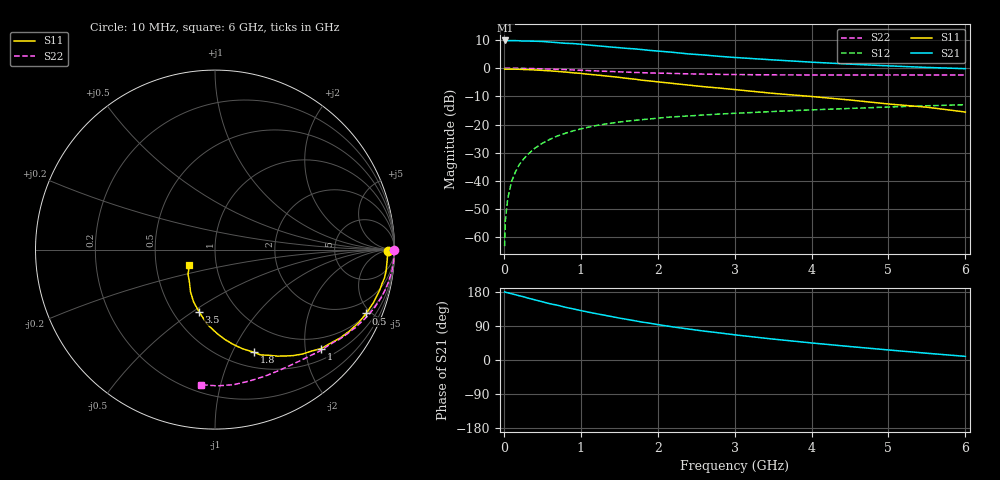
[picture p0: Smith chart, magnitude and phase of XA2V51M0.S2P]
! SIEMENS Discrete & RF Semiconductors
! BFY180
! Si NPN RF Bipolar Junction Transistor in MICRO-X
! VCE = 2.5 V  IC = 1 mA
! Common Emitter S-Parameters:  May  1997
# GHz  S  MA  R  50
!  f  S11  S21  S12  S22
! GHz  MAG  ANG  MAG  ANG  MAG  ANG  MAG  ANG
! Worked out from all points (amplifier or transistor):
!   36 points, 10 MHz to 6 GHz, reference 50 ohm
!   highest |S21| = 9.8 dB at 20 MHz (marker M1)
!   |S21| within 3 dB of that: start of sweep to 1.709 GHz
!   unconditionally stable (mu >= 1): 3.756 GHz to end of sweep
!   at 250 MHz: K = 0.07, MSG = 21.0 dB, |S12| = -32.4 dB
!   at 1.4 GHz: K = 0.52, MSG = 13.5 dB, |S12| = -19.5 dB
!   at 6 GHz: K = 1.07, MAG = 4.8 dB, |S12| = -12.9 dB
!   S11 on the Smith chart (normalised r, x): 10 MHz: 51, -9; 500 MHz: 1.08, -4.70; 1 GHz: 0.73, -2.34; 1.8 GHz: 0.66, -1.22; 3.5 GHz: 0.67, -0.53; 6 GHz: 0.74, -0.13
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0.01  0.963 -0.4  3.058 179.6  0.0007 90.9  0.9984 -0.2
0.02  0.9608 -0.9  3.103 178.8  0.002 91.9  0.9999 -0.6
0.05  0.9618 -2.0  3.077 177.5  0.0048 87.2  0.9974 -1.3
0.1  0.961 -4.3  3.083 174.9  0.0098 88.8  0.9975 -2.8
0.15  0.9605 -7.1  3.078 172.3  0.0144 86.5  0.9966 -4.1
0.2  0.9575 -9.4  3.063 169.5  0.0195 83.2  0.9941 -5.4
0.3  0.9455 -13.7  3.029 164.2  0.0286 80.7  0.9891 -8.1
0.5  0.9144 -22.9  2.981 153.7  0.0466 73.8  0.9743 -13.3
0.6  0.8977 -26.9  2.906 148.4  0.055 71.1  0.9656 -15.7
0.7  0.876 -31.2  2.838 144.4  0.0632 68.4  0.9547 -18.1
0.8  0.8538 -35.2  2.763 139.2  0.0703 65.8  0.9433 -20.4
1  0.8087 -43.0  2.662 130.5  0.084 60.4  0.9191 -24.8
1.1  0.7814 -46.3  2.575 126.3  0.0901 57.7  0.9063 -26.8
1.5  0.6875 -59.7  2.309 110.7  0.1111 49.7  0.8622 -34.4
1.8  0.6118 -69.3  2.134 100.0  0.1227 45.2  0.8328 -39.2
2.2  0.5365 -79.3  1.911 87.3  0.1372 39.6  0.8072 -45.3
2.6  0.4698 -88.3  1.715 76.3  0.1482 35.6  0.7858 -50.7
3  0.4183 -96.0  1.55 66.5  0.1586 31.6  0.7717 -55.9
3.5  0.3581 -104.3  1.404 55.2  0.1707 27.7  0.762 -62.2
4.5  0.2729 -120.0  1.181 35.5  0.1937 19.9  0.7568 -75.2
5.5  0.2035 -137.5  1.032 17.8  0.2157 12.1  0.7594 -89.0
6  0.167 -149.0  0.981 9.6  0.2252 7.9  0.7567 -96.0
